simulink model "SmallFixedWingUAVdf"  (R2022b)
settings: Solver=ode4  StartTime=0  StopTime=stoptime  FixedStep=0.001  RelTol=1e-3  EnableMultiTasking=on
PreLoadFcn:
  | asbswarm_vehicledata; % load in workspace variables
PostLoadFcn:
  | open_system([gcs,'/MATLAB Animation Display/MATLAB',10,'Animation']);
InitFcn:
  | InitDatactrl
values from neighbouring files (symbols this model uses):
  env = struct    [InitDatactrl.m]
  F = Fattr + Frep    [APF.m]
  q = ix-1    [bspline_deboor.m]
  SenorSampleTime = 0.01    [InitDatactrl.m]
  sensors = struct    [InitDatactrl.m]
  uav = struct    [InitDatactrl.m]    (also in InitDatactrldf.m)
undefined symbols (not defined in the file or in its folder): Busy, Continuous, DiscIntNeverNeededParam, Dryden, Earth, Light, MIL, Newton, pa28, r, Raphson, sigbuilder_block, Wait, WGS84
libraries: simulink x37, aerolibactuator x10, sharedtransform x6, aerolibatmos2 x4, aerolibasang x4, aerolibwind2 x4, aerolibtransform2 x3, aerolibconvert2 x3, aerolibfltsims x2, shared6dof x2, aerolibnav x2, aerolibanimutils x1
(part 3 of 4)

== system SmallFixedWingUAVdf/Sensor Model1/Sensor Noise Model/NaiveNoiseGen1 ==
  Signal In : Inport
  Noise On : Inport  Port=2
  Add : Sum
  Band-Limited White Noise : simulink/Sources/Band-Limited White Noise  Cov=np  Ts=st  seed=ns
  Gain : Gain  Gain=ng
  Switch : Switch  Threshold=0.3
  Signal Out : Outport  VectorParamsAs1DForOutWhenUnconnected=off
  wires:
  Gain/1 -> Add/2
  Signal In/1 -> Add/1, Switch/3
  Switch/1 -> Signal Out/1
  Noise On/1 -> Switch/2
  Add/1 -> Switch/1
  Band-Limited White Noise/1 -> Gain/1

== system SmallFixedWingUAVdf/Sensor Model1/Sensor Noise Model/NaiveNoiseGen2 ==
  Signal In : Inport
  Noise On : Inport  Port=2
  Add : Sum
  Band-Limited White Noise : simulink/Sources/Band-Limited White Noise  Cov=np  Ts=st  seed=ns
  Gain : Gain  Gain=ng
  Switch : Switch  Threshold=0.3
  Signal Out : Outport  VectorParamsAs1DForOutWhenUnconnected=off
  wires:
  Gain/1 -> Add/2
  Signal In/1 -> Add/1, Switch/3
  Switch/1 -> Signal Out/1
  Noise On/1 -> Switch/2
  Add/1 -> Switch/1
  Band-Limited White Noise/1 -> Gain/1

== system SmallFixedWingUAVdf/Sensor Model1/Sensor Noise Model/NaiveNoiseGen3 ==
  Signal In : Inport
  Noise On : Inport  Port=2
  Add : Sum
  Band-Limited White Noise : simulink/Sources/Band-Limited White Noise  Cov=np  Ts=st  seed=ns
  Gain : Gain  Gain=ng
  Switch : Switch  Threshold=0.3
  Signal Out : Outport  VectorParamsAs1DForOutWhenUnconnected=off
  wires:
  Gain/1 -> Add/2
  Signal In/1 -> Add/1, Switch/3
  Switch/1 -> Signal Out/1
  Noise On/1 -> Switch/2
  Add/1 -> Switch/1
  Band-Limited White Noise/1 -> Gain/1

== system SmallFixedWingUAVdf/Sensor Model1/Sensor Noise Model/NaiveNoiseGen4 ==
  Signal In : Inport
  Noise On : Inport  Port=2
  Add : Sum
  Band-Limited White Noise : simulink/Sources/Band-Limited White Noise  Cov=np  Ts=st  seed=ns
  Gain : Gain  Gain=ng
  Switch : Switch  Threshold=0.3
  Signal Out : Outport  VectorParamsAs1DForOutWhenUnconnected=off
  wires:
  Gain/1 -> Add/2
  Signal In/1 -> Add/1, Switch/3
  Switch/1 -> Signal Out/1
  Noise On/1 -> Switch/2
  Add/1 -> Switch/1
  Band-Limited White Noise/1 -> Gain/1

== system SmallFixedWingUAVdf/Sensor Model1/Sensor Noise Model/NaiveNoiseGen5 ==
  Signal In : Inport
  Noise On : Inport  Port=2
  Add : Sum
  Band-Limited White Noise : simulink/Sources/Band-Limited White Noise  Cov=np  Ts=st  seed=ns
  Gain : Gain  Gain=ng
  Switch : Switch  Threshold=0.3
  Signal Out : Outport  VectorParamsAs1DForOutWhenUnconnected=off
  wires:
  Gain/1 -> Add/2
  Signal In/1 -> Add/1, Switch/3
  Switch/1 -> Signal Out/1
  Noise On/1 -> Switch/2
  Add/1 -> Switch/1
  Band-Limited White Noise/1 -> Gain/1

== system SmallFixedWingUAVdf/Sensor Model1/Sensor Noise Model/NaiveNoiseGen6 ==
  Signal In : Inport
  Noise On : Inport  Port=2
  Add : Sum
  Band-Limited White Noise : simulink/Sources/Band-Limited White Noise  Cov=np  Ts=st  seed=ns
  Gain : Gain  Gain=ng
  Switch : Switch  Threshold=0.3
  Signal Out : Outport  VectorParamsAs1DForOutWhenUnconnected=off
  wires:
  Gain/1 -> Add/2
  Signal In/1 -> Add/1, Switch/3
  Switch/1 -> Signal Out/1
  Noise On/1 -> Switch/2
  Add/1 -> Switch/1
  Band-Limited White Noise/1 -> Gain/1

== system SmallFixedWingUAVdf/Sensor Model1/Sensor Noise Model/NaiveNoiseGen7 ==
  Signal In : Inport
  Noise On : Inport  Port=2
  Add : Sum
  Band-Limited White Noise : simulink/Sources/Band-Limited White Noise  Cov=np  Ts=st  seed=ns
  Gain : Gain  Gain=ng
  Switch : Switch  Threshold=0.3
  Signal Out : Outport  VectorParamsAs1DForOutWhenUnconnected=off
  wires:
  Gain/1 -> Add/2
  Signal In/1 -> Add/1, Switch/3
  Switch/1 -> Signal Out/1
  Noise On/1 -> Switch/2
  Add/1 -> Switch/1
  Band-Limited White Noise/1 -> Gain/1

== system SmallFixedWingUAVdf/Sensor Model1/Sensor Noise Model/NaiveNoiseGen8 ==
  Signal In : Inport
  Noise On : Inport  Port=2
  Add : Sum
  Band-Limited White Noise : simulink/Sources/Band-Limited White Noise  Cov=np  Ts=st  seed=ns
  Gain : Gain  Gain=ng
  Switch : Switch  Threshold=0.3
  Signal Out : Outport  VectorParamsAs1DForOutWhenUnconnected=off
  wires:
  Gain/1 -> Add/2
  Signal In/1 -> Add/1, Switch/3
  Switch/1 -> Signal Out/1
  Noise On/1 -> Switch/2
  Add/1 -> Switch/1
  Band-Limited White Noise/1 -> Gain/1

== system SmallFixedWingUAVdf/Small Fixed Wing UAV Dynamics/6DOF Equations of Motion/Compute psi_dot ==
  Euler : Inport
  G : Inport  Port=2
  Mux1 : Mux  Inputs=2
  psidot : Fcn  Expr=(u[5]*sin(u[1])+u[6]*cos(u[1]))/cos(u[2])
  psi_dot : Outport  Unit=rad/S  VectorParamsAs1DForOutWhenUnconnected=off
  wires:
  G/1 -> Mux1/2
  psidot/1 -> psi_dot/1  "psi_dot"
  Mux1/1 -> psidot/1
  Euler/1 -> Mux1/1

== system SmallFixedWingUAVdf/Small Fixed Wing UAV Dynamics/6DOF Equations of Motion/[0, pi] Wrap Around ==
  Euler : Inport
  Compare To Zero : simulink/Logic and Bit Operations/Compare To Zero  relop=>=  OutDataTypeStr=uint8  ZeroCross=off
  Logical Operator : Logic  Operator=NOT  AllPortsSameDT=off  OutDataTypeStr=boolean
  Merge : Merge  InitialOutput=0
  Mux2 : Mux  Inputs=2
  Negative Yaw : Subsystem
  Positive Yaw : Subsystem
  Selector1 : Selector  InputPortWidth=3  IndexOptions=Index vector (dialog)  Indices=[1 2]  OutputSizes=1
  Selector2 : Selector  InputPortWidth=3  IndexOptions=Index vector (dialog)  Indices=[3]  OutputSizes=1
  Wrapped : Outport  VectorParamsAs1DForOutWhenUnconnected=off
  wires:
  Negative Yaw/1(yaw_wr) -> Merge/2
  Positive Yaw/1(yaw_wr) -> Merge/1
  Merge/1 -> Mux2/2
  Logical Operator/1 -> Negative Yaw/Enable
  Compare To Zero/1 -> Logical Operator/1, Positive Yaw/Enable
  Selector2/1 -> Negative Yaw/1(yaw), Positive Yaw/1(yaw), Compare To Zero/1
  Mux2/1 -> Wrapped/1
  Selector1/1 -> Mux2/1
  Euler/1 -> Selector1/1, Selector2/1

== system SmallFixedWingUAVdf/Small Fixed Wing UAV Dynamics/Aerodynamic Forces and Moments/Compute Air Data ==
  Vb : Inport  PortDimensions=3
  Rho : Inport  Port=2
  Bus Creator : BusCreator  Inputs=4
  Dynamic Pressure : aerolibasang/Dynamic Pressure
  "Incidence, Sideslip, & Airspeed" : aerolibasang/Incidence, Sideslip, & Airspeed
  AirData : Outport  VectorParamsAs1DForOutWhenUnconnected=off
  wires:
  Bus Creator/1 -> AirData/1
  "Incidence, Sideslip, & Airspeed"/1 -> Bus Creator/1  "alpha"
  Rho/1 -> Dynamic Pressure/2
  "Incidence, Sideslip, & Airspeed"/3 -> Bus Creator/3  "airpseed"
  Dynamic Pressure/1 -> Bus Creator/4  "q"
  Vb/1 -> "Incidence, Sideslip, & Airspeed"/1, Dynamic Pressure/1
  "Incidence, Sideslip, & Airspeed"/2 -> Bus Creator/2  "beta"

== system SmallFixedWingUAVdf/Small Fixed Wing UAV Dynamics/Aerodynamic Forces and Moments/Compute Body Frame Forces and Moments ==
  AirData : Inport
  CtrlSurfaces : Inport  Port=2
  p,q,r : Inport  Port=3
  Bus Selector : BusSelector  OutputSignals=alpha,beta
  Mux : Mux  Inputs=2
  Rotate FM to body frame : Subsystem
  Wind frame F& M : Subsystem
  F_b : Outport  Unit=kg*m/s^2  VectorParamsAs1DForOutWhenUnconnected=off
  M_b : Outport  Port=2  Unit=kg*m/s  VectorParamsAs1DForOutWhenUnconnected=off
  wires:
  Mux/1 -> Rotate FM to body frame/2(alpha_beta)
  Bus Selector/2 -> Mux/2  "<beta>"
  Bus Selector/1 -> Mux/1  "<alpha>"
  Wind frame F& M/1(FM_w) -> Rotate FM to body frame/1(FM_w)  "FM_W"
  p,q,r/1 -> Wind frame F& M/3(p,q,r)
  Rotate FM to body frame/2(M_b) -> M_b/1
  Rotate FM to body frame/1(F_b) -> F_b/1
  CtrlSurfaces/1 -> Wind frame F& M/2(CtrlSurfaces)
  AirData/1 -> Wind frame F& M/1(Airdata), Bus Selector/1

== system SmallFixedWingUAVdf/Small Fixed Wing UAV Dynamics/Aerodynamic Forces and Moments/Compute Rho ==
  Xe : Inport
  Gain : Gain  Gain=-1
  Get Z : Selector  InputPortWidth=3  IndexOptions=Index vector (dialog)  Indices=[3]  OutputSizes=[(-2)]
  ISA Atmosphere Model1 : aerolibatmos2/ISA Atmosphere Model  custom=on  g=env.ISA_g  gamma=1.4  R=env.ISA_R  L=env.ISA_lapse  h_trop=11000  h_strat=20000  rho0=env.ISA_rho0  P0=env.ISA_P0  T0=env.ISA_T0  h0=0
  Terminator : Terminator
  Terminator1 : Terminator
  Terminator2 : Terminator
  Transfer Fcn : TransferFcn  Denominator=[.01 1]
  Rho : Outport  VectorParamsAs1DForOutWhenUnconnected=off
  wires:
  ISA Atmosphere Model1/2 -> Terminator1/1
  ISA Atmosphere Model1/1 -> Terminator/1  "OAT"
  Gain/1 -> ISA Atmosphere Model1/1
  Get Z/1 -> Transfer Fcn/1
  Transfer Fcn/1 -> Gain/1
  ISA Atmosphere Model1/3 -> Terminator2/1  "static"
  Xe/1 -> Get Z/1
  ISA Atmosphere Model1/4 -> Rho/1

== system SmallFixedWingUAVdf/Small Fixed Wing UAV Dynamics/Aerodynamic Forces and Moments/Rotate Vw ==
  Vw : Inport
  Euler : Inport  Port=2
  RL2B : Subsystem
  RL2B * Vw : Product  Multiplication=Matrix(*)  InputSameDT=on  SaturateOnIntegerOverflow=on
  Vb : Outport  Unit=m/s  VectorParamsAs1DForOutWhenUnconnected=off
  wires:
  RL2B * Vw/1 -> Vb/1
  Vw/1 -> RL2B * Vw/2
  RL2B/1(RL2B) -> RL2B * Vw/1
  Euler/1 -> RL2B/1(Euler)

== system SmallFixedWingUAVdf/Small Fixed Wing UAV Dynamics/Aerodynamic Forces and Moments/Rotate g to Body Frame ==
  Euler : Inport
  Gravity Force : Inport  Port=2  PortDimensions=3
  Product1 : Product  Multiplication=Matrix(*)  InputSameDT=on  SaturateOnIntegerOverflow=on
  RL2B : Subsystem
  g_b : Outport  Unit=kg*m/s^2  VectorParamsAs1DForOutWhenUnconnected=off
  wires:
  Gravity Force/1 -> Product1/2
  Euler/1 -> RL2B/1(Euler)
  Product1/1 -> g_b/1
  RL2B/1(RL2B) -> Product1/1

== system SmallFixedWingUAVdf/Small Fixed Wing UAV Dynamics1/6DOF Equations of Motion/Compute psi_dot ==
  Euler : Inport
  G : Inport  Port=2
  Mux1 : Mux  Inputs=2
  psidot : Fcn  Expr=(u[5]*sin(u[1])+u[6]*cos(u[1]))/cos(u[2])
  psi_dot : Outport  Unit=rad/S  VectorParamsAs1DForOutWhenUnconnected=off
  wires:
  G/1 -> Mux1/2
  psidot/1 -> psi_dot/1  "psi_dot"
  Mux1/1 -> psidot/1
  Euler/1 -> Mux1/1

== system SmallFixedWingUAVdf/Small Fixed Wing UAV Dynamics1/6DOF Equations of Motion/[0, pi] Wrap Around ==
  Euler : Inport
  Compare To Zero : simulink/Logic and Bit Operations/Compare To Zero  relop=>=  OutDataTypeStr=uint8  ZeroCross=off
  Logical Operator : Logic  Operator=NOT  AllPortsSameDT=off  OutDataTypeStr=boolean
  Merge : Merge  InitialOutput=0
  Mux2 : Mux  Inputs=2
  Negative Yaw : Subsystem
  Positive Yaw : Subsystem
  Selector1 : Selector  InputPortWidth=3  IndexOptions=Index vector (dialog)  Indices=[1 2]  OutputSizes=1
  Selector2 : Selector  InputPortWidth=3  IndexOptions=Index vector (dialog)  Indices=[3]  OutputSizes=1
  Wrapped : Outport  VectorParamsAs1DForOutWhenUnconnected=off
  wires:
  Negative Yaw/1(yaw_wr) -> Merge/2
  Positive Yaw/1(yaw_wr) -> Merge/1
  Merge/1 -> Mux2/2
  Logical Operator/1 -> Negative Yaw/Enable
  Compare To Zero/1 -> Logical Operator/1, Positive Yaw/Enable
  Selector2/1 -> Negative Yaw/1(yaw), Positive Yaw/1(yaw), Compare To Zero/1
  Mux2/1 -> Wrapped/1
  Selector1/1 -> Mux2/1
  Euler/1 -> Selector1/1, Selector2/1

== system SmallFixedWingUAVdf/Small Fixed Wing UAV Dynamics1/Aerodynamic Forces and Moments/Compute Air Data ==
  Vb : Inport  PortDimensions=3
  Rho : Inport  Port=2
  Bus Creator : BusCreator  Inputs=4
  Dynamic Pressure : aerolibasang/Dynamic Pressure
  "Incidence, Sideslip, & Airspeed" : aerolibasang/Incidence, Sideslip, & Airspeed
  AirData : Outport  VectorParamsAs1DForOutWhenUnconnected=off
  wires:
  Bus Creator/1 -> AirData/1  "AirData"
  "Incidence, Sideslip, & Airspeed"/1 -> Bus Creator/1  "alpha"
  Rho/1 -> Dynamic Pressure/2
  "Incidence, Sideslip, & Airspeed"/3 -> Bus Creator/3  "airpseed"
  Dynamic Pressure/1 -> Bus Creator/4  "q"
  Vb/1 -> "Incidence, Sideslip, & Airspeed"/1, Dynamic Pressure/1
  "Incidence, Sideslip, & Airspeed"/2 -> Bus Creator/2  "beta"

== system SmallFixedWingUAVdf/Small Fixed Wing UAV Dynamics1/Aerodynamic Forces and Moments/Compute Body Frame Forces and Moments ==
  AirData : Inport
  CtrlSurfaces : Inport  Port=2
  p,q,r : Inport  Port=3
  Bus Selector : BusSelector  OutputSignals=alpha,beta
  Mux : Mux  Inputs=2
  Rotate FM to body frame : Subsystem
  Wind frame F& M : Subsystem
  F_b : Outport  Unit=kg*m/s^2  VectorParamsAs1DForOutWhenUnconnected=off
  M_b : Outport  Port=2  Unit=kg*m/s  VectorParamsAs1DForOutWhenUnconnected=off
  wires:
  Mux/1 -> Rotate FM to body frame/2(alpha_beta)
  Bus Selector/2 -> Mux/2  "<beta>"
  Bus Selector/1 -> Mux/1  "<alpha>"
  Wind frame F& M/1(FM_w) -> Rotate FM to body frame/1(FM_w)  "FM_W"
  p,q,r/1 -> Wind frame F& M/3(p,q,r)
  Rotate FM to body frame/2(M_b) -> M_b/1
  Rotate FM to body frame/1(F_b) -> F_b/1
  CtrlSurfaces/1 -> Wind frame F& M/2(CtrlSurfaces)
  AirData/1 -> Wind frame F& M/1(Airdata), Bus Selector/1

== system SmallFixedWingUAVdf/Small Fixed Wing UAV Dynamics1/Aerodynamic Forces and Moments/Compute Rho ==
  Xe : Inport
  Gain : Gain  Gain=-1
  Get Z : Selector  InputPortWidth=3  IndexOptions=Index vector (dialog)  Indices=[3]  OutputSizes=[(-2)]
  ISA Atmosphere Model1 : aerolibatmos2/ISA Atmosphere Model  custom=on  g=env.ISA_g  gamma=1.4  R=env.ISA_R  L=env.ISA_lapse  h_trop=11000  h_strat=20000  rho0=env.ISA_rho0  P0=env.ISA_P0  T0=env.ISA_T0  h0=0
  Terminator : Terminator
  Terminator1 : Terminator
  Terminator2 : Terminator
  Transfer Fcn : TransferFcn  Denominator=[.01 1]
  Rho : Outport  VectorParamsAs1DForOutWhenUnconnected=off
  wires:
  ISA Atmosphere Model1/2 -> Terminator1/1
  ISA Atmosphere Model1/1 -> Terminator/1  "OAT"
  Gain/1 -> ISA Atmosphere Model1/1
  Get Z/1 -> Transfer Fcn/1
  Transfer Fcn/1 -> Gain/1
  ISA Atmosphere Model1/3 -> Terminator2/1  "static"
  Xe/1 -> Get Z/1
  ISA Atmosphere Model1/4 -> Rho/1

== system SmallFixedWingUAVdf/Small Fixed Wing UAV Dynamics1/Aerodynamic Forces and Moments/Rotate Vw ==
  Vw : Inport
  Euler : Inport  Port=2
  RL2B : Subsystem
  RL2B * Vw : Product  Multiplication=Matrix(*)  InputSameDT=on  SaturateOnIntegerOverflow=on
  Vb : Outport  Unit=m/s  VectorParamsAs1DForOutWhenUnconnected=off
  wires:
  RL2B * Vw/1 -> Vb/1
  Vw/1 -> RL2B * Vw/2
  RL2B/1(RL2B) -> RL2B * Vw/1
  Euler/1 -> RL2B/1(Euler)

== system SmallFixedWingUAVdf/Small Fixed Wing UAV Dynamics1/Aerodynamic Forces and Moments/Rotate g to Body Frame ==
  Euler : Inport
  Gravity Force : Inport  Port=2  PortDimensions=3
  Product1 : Product  Multiplication=Matrix(*)  InputSameDT=on  SaturateOnIntegerOverflow=on
  RL2B : Subsystem
  g_b : Outport  Unit=kg*m/s^2  VectorParamsAs1DForOutWhenUnconnected=off
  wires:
  Gravity Force/1 -> Product1/2
  Euler/1 -> RL2B/1(Euler)
  Product1/1 -> g_b/1
  RL2B/1(RL2B) -> Product1/1

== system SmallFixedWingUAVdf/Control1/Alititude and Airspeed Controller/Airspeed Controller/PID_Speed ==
  x : Inport
  reset_i : Inport  Port=2
  Derivative Gain : Gain  DisableCoverage=on  Gain=0  ParamMin=-100  ParamMax=100  OutMin=-100  OutMax=100
  Discrete Derivative : simulink/Discrete/Discrete Derivative  gainval=1.0  ICPrevScaledInput=0.0  OutMin=[]  OutMax=[]  OutDataType=fixdt(1, 16)  OutScaling=2^-10  DoSatur=off
  Discrete-Time Integrator : DiscreteIntegrator  ExternalReset=either  SampleTime=-1  UpperSaturationLimit=0.3  LowerSaturationLimit=-0.3  ICPrevOutput=DiscIntNeverNeededParam  ICPrevScaledInput=DiscIntNeverNeededParam
  Gain : Gain  Gain=0.5
  Integral Gain : Gain  DisableCoverage=on  Gain=0.13
  Sum : Sum  Inputs=+++
  y : Outport  InitialOutput=0  VectorParamsAs1DForOutWhenUnconnected=off
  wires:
  reset_i/1 -> Discrete-Time Integrator/2
  Discrete-Time Integrator/1 -> Sum/2
  Discrete Derivative/1 -> Sum/3
  Sum/1 -> y/1
  Gain/1 -> Sum/1
  Derivative Gain/1 -> Discrete Derivative/1
  Integral Gain/1 -> Discrete-Time Integrator/1
  x/1 -> Derivative Gain/1, Integral Gain/1, Gain/1

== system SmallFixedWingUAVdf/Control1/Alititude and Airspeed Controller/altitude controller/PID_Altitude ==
  x : Inport
  reset_i : Inport  Port=2
  Derivative Gain : Gain  DisableCoverage=on  Gain=0  ParamMin=-100  ParamMax=100  OutMin=-100  OutMax=100
  Discrete Derivative : simulink/Discrete/Discrete Derivative  gainval=1.0  ICPrevScaledInput=0.0  OutMin=[]  OutMax=[]  OutDataType=fixdt(1, 16)  OutScaling=2^-10  DoSatur=off
  Discrete-Time Integrator : DiscreteIntegrator  ExternalReset=either  SampleTime=-1  ICPrevOutput=DiscIntNeverNeededParam  ICPrevScaledInput=DiscIntNeverNeededParam
  Gain : Gain  Gain=0.055
  Integral Gain : Gain  DisableCoverage=on  Gain=0
  Sum : Sum  Inputs=+++
  y : Outport  InitialOutput=0  VectorParamsAs1DForOutWhenUnconnected=off
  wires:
  x/1 -> Gain/1, Integral Gain/1, Derivative Gain/1
  Integral Gain/1 -> Discrete-Time Integrator/1
  Derivative Gain/1 -> Discrete Derivative/1
  Gain/1 -> Sum/1
  Sum/1 -> y/1
  Discrete Derivative/1 -> Sum/3
  Discrete-Time Integrator/1 -> Sum/2
  reset_i/1 -> Discrete-Time Integrator/2

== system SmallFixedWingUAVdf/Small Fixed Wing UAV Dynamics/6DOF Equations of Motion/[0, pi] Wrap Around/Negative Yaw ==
  yaw : Inport
  Enable : EnablePort
  Abs : Abs
  Constant1 : Constant  Value=2*pi
  Constant2 : Constant  Value=2*pi
  Math Function : Math  Operator=mod  SignedPower=on
  Sum : Sum  Inputs=|-+
  yaw_wr : Outport  VectorParamsAs1DForOutWhenUnconnected=off
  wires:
  Sum/1 -> yaw_wr/1
  Constant2/1 -> Sum/2
  Abs/1 -> Math Function/1
  Math Function/1 -> Sum/1
  Constant1/1 -> Math Function/2
  yaw/1 -> Abs/1

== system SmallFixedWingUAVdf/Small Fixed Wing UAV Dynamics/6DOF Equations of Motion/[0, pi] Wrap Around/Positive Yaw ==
  yaw : Inport
  Enable : EnablePort
  Constant1 : Constant  Value=2*pi
  Math Function : Math  Operator=mod  SignedPower=on
  yaw_wr : Outport  VectorParamsAs1DForOutWhenUnconnected=off
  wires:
  Math Function/1 -> yaw_wr/1
  Constant1/1 -> Math Function/2
  yaw/1 -> Math Function/1

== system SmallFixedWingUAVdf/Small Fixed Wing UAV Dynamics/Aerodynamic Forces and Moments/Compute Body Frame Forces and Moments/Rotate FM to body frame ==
  FM_w : Inport
  alpha_beta : Inport  Port=2
  Forces : Selector  InputPortWidth=6  IndexOptions=Index vector (dialog)  Indices=[1 2 3]  OutputSizes=[(-2)]
  Moments : Selector  InputPortWidth=6  IndexOptions=Index vector (dialog)  Indices=[4 5 6]  OutputSizes=[(-2)]
  Rotate Forces : Subsystem
  Rotate Moments : Subsystem
  F_b : Outport  VectorParamsAs1DForOutWhenUnconnected=off
  M_b : Outport  Port=2  VectorParamsAs1DForOutWhenUnconnected=off
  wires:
  alpha_beta/1 -> Rotate Forces/2(alpha_beta), Rotate Moments/1(alpha_beta)
  Moments/1 -> Rotate Moments/2(M_w)
  FM_w/1 -> Moments/1, Forces/1
  Forces/1 -> Rotate Forces/1(F_w)
  Rotate Moments/1(M_b) -> M_b/1
  Rotate Forces/1(F_b) -> F_b/1

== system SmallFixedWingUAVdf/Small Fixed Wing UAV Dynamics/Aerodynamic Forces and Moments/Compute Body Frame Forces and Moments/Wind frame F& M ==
  Airdata : Inport
  CtrlSurfaces : Inport  Port=2
  p,q,r : Inport  Port=3
  Bus Creator1 : BusCreator  Inputs=2
  Bus Selector1 : BusSelector  OutputSignals=dA,dR
  Bus Selector2 : BusSelector  OutputSignals=dE,dF
  Bus Selector6 : BusSelector  OutputSignals=beta,airpseed
  Bus Selector7 : BusSelector  OutputSignals=alpha,airpseed
  Get Forces and Moments : Subsystem
  Lateral Channel : Subsystem
  Longitudinal Channel : Subsystem
  FM_w : Outport  PortDimensions=6  VectorParamsAs1DForOutWhenUnconnected=off
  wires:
  Get Forces and Moments/1(FM_w) -> FM_w/1
  Bus Creator1/1 -> Get Forces and Moments/2(AeroCoeffs)
  Bus Selector7/2 -> Longitudinal Channel/2(Airpseed)  "<airpseed>"
  Bus Selector7/1 -> Longitudinal Channel/1(alpha)  "<alpha>"
  Bus Selector6/2 -> Lateral Channel/2(Airspeed)  "<airpseed>"
  Bus Selector6/1 -> Lateral Channel/1(beta)  "<beta>"
  Airdata/1 -> Bus Selector6/1, Bus Selector7/1, Get Forces and Moments/1(Airdata)
  Bus Selector2/2 -> Longitudinal Channel/4(dF)  "<dF>"
  Bus Selector2/1 -> Longitudinal Channel/3(dE)  "<dE>"
  Bus Selector1/2 -> Lateral Channel/4(dR)  "<dR>"
  Bus Selector1/1 -> Lateral Channel/3(dA)  "<dA>"
  CtrlSurfaces/1 -> Bus Selector1/1, Bus Selector2/1
  p,q,r/1 -> Lateral Channel/5(p,q,r), Longitudinal Channel/5(p,q,r)
  Lateral Channel/1(Lateral) -> Bus Creator1/1
  Longitudinal Channel/1(Longitudinal) -> Bus Creator1/2

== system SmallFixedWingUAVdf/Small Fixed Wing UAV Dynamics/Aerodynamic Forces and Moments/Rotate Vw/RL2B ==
  Euler : Inport
  Rotation Angles to Direction Cosine Matrix : sharedtransform/Rotation Angles to Direction Cosine Matrix  rotationOrder=ZYX  aMode=aMode
  Selector : Selector  InputPortWidth=3  IndexOptions=Index vector (dialog)  Indices=[3 2 1]  OutputSizes=1
  RL2B : Outport  VectorParamsAs1DForOutWhenUnconnected=off
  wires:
  Rotation Angles to Direction Cosine Matrix/1 -> RL2B/1
  Euler/1 -> Selector/1
  Selector/1 -> Rotation Angles to Direction Cosine Matrix/1

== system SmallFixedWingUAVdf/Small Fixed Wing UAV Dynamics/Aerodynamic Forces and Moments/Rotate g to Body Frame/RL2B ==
  Euler : Inport
  Rotation Angles to Direction Cosine Matrix : sharedtransform/Rotation Angles to Direction Cosine Matrix  rotationOrder=ZYX  aMode=aMode
  Selector : Selector  InputPortWidth=3  IndexOptions=Index vector (dialog)  Indices=[3 2 1]  OutputSizes=1
  RL2B : Outport  VectorParamsAs1DForOutWhenUnconnected=off
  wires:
  Rotation Angles to Direction Cosine Matrix/1 -> RL2B/1
  Euler/1 -> Selector/1
  Selector/1 -> Rotation Angles to Direction Cosine Matrix/1

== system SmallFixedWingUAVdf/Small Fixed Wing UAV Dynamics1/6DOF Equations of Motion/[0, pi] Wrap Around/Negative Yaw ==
  yaw : Inport
  Enable : EnablePort
  Abs : Abs
  Constant1 : Constant  Value=2*pi
  Constant2 : Constant  Value=2*pi
  Math Function : Math  Operator=mod  SignedPower=on
  Sum : Sum  Inputs=|-+
  yaw_wr : Outport  VectorParamsAs1DForOutWhenUnconnected=off
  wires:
  Sum/1 -> yaw_wr/1
  Constant2/1 -> Sum/2
  Abs/1 -> Math Function/1
  Math Function/1 -> Sum/1
  Constant1/1 -> Math Function/2
  yaw/1 -> Abs/1

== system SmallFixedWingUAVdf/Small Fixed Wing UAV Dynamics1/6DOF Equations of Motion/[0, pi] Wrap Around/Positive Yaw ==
  yaw : Inport
  Enable : EnablePort
  Constant1 : Constant  Value=2*pi
  Math Function : Math  Operator=mod  SignedPower=on
  yaw_wr : Outport  VectorParamsAs1DForOutWhenUnconnected=off
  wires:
  Math Function/1 -> yaw_wr/1
  Constant1/1 -> Math Function/2
  yaw/1 -> Math Function/1

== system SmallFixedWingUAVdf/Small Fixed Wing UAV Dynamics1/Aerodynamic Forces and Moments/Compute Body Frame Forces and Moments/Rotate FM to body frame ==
  FM_w : Inport
  alpha_beta : Inport  Port=2
  Forces : Selector  InputPortWidth=6  IndexOptions=Index vector (dialog)  Indices=[1 2 3]  OutputSizes=[(-2)]
  Moments : Selector  InputPortWidth=6  IndexOptions=Index vector (dialog)  Indices=[4 5 6]  OutputSizes=[(-2)]
  Rotate Forces : Subsystem
  Rotate Moments : Subsystem
  F_b : Outport  VectorParamsAs1DForOutWhenUnconnected=off
  M_b : Outport  Port=2  VectorParamsAs1DForOutWhenUnconnected=off
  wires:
  alpha_beta/1 -> Rotate Forces/2(alpha_beta), Rotate Moments/1(alpha_beta)
  Moments/1 -> Rotate Moments/2(M_w)
  FM_w/1 -> Moments/1, Forces/1
  Forces/1 -> Rotate Forces/1(F_w)
  Rotate Moments/1(M_b) -> M_b/1
  Rotate Forces/1(F_b) -> F_b/1

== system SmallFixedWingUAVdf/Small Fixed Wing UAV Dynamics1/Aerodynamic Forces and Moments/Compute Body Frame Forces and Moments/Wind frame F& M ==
  Airdata : Inport
  CtrlSurfaces : Inport  Port=2
  p,q,r : Inport  Port=3
  Bus Creator1 : BusCreator  Inputs=2
  Bus Selector1 : BusSelector  OutputSignals=dA,dR
  Bus Selector2 : BusSelector  OutputSignals=dE,dF
  Bus Selector6 : BusSelector  OutputSignals=beta,airpseed
  Bus Selector7 : BusSelector  OutputSignals=alpha,airpseed
  Get Forces and Moments : Subsystem
  Lateral Channel : Subsystem
  Longitudinal Channel : Subsystem
  FM_w : Outport  PortDimensions=6  VectorParamsAs1DForOutWhenUnconnected=off
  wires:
  Get Forces and Moments/1(FM_w) -> FM_w/1
  Bus Creator1/1 -> Get Forces and Moments/2(AeroCoeffs)
  Bus Selector7/2 -> Longitudinal Channel/2(Airpseed)  "<airpseed>"
  Bus Selector7/1 -> Longitudinal Channel/1(alpha)  "<alpha>"
  Bus Selector6/2 -> Lateral Channel/2(Airspeed)  "<airpseed>"
  Bus Selector6/1 -> Lateral Channel/1(beta)  "<beta>"
  Airdata/1 -> Get Forces and Moments/1(Airdata), Bus Selector7/1, Bus Selector6/1
  Bus Selector2/2 -> Longitudinal Channel/4(dF)  "<dF>"
  Bus Selector2/1 -> Longitudinal Channel/3(dE)  "<dE>"
  Bus Selector1/2 -> Longitudinal Channel/6(dR), Lateral Channel/4(dR)  "<dR>"
  Bus Selector1/1 -> Lateral Channel/3(dA)  "<dA>"
  CtrlSurfaces/1 -> Bus Selector2/1, Bus Selector1/1
  p,q,r/1 -> Lateral Channel/5(p,q,r), Longitudinal Channel/5(p,q,r)
  Lateral Channel/1(Lateral) -> Bus Creator1/1
  Longitudinal Channel/1(Longitudinal) -> Bus Creator1/2

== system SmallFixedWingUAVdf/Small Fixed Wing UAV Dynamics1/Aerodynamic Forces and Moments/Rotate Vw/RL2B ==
  Euler : Inport
  Rotation Angles to Direction Cosine Matrix : sharedtransform/Rotation Angles to Direction Cosine Matrix  rotationOrder=ZYX  aMode=aMode
  Selector : Selector  InputPortWidth=3  IndexOptions=Index vector (dialog)  Indices=[3 2 1]  OutputSizes=1
  RL2B : Outport  VectorParamsAs1DForOutWhenUnconnected=off
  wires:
  Rotation Angles to Direction Cosine Matrix/1 -> RL2B/1
  Euler/1 -> Selector/1
  Selector/1 -> Rotation Angles to Direction Cosine Matrix/1

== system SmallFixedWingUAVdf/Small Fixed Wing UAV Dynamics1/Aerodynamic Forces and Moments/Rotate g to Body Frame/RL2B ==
  Euler : Inport
  Rotation Angles to Direction Cosine Matrix : sharedtransform/Rotation Angles to Direction Cosine Matrix  rotationOrder=ZYX  aMode=aMode
  Selector : Selector  InputPortWidth=3  IndexOptions=Index vector (dialog)  Indices=[3 2 1]  OutputSizes=1
  RL2B : Outport  VectorParamsAs1DForOutWhenUnconnected=off
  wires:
  Rotation Angles to Direction Cosine Matrix/1 -> RL2B/1
  Euler/1 -> Selector/1
  Selector/1 -> Rotation Angles to Direction Cosine Matrix/1

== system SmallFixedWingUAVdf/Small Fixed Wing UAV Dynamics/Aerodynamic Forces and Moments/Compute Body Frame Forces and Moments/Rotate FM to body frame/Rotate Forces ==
  F_w : Inport
  alpha_beta : Inport  Port=2
  Product2 : Product  Multiplication=Matrix(*)  SaturateOnIntegerOverflow=on
  RB2W : Subsystem
  RW2B : Math  Operator=transpose  SignedPower=on
  F_b : Outport  PortDimensions=3  VectorParamsAs1DForOutWhenUnconnected=off
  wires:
  RW2B/1 -> Product2/1
  F_w/1 -> Product2/2
  Product2/1 -> F_b/1
  alpha_beta/1 -> RB2W/1(aoa beta)
  RB2W/1(Rw2b) -> RW2B/1

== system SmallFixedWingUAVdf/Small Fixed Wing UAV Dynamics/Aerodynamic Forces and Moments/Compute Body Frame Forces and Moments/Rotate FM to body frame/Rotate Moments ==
  alpha_beta : Inport
  M_w : Inport  Port=2
  Product2 : Product  Multiplication=Matrix(*)  SaturateOnIntegerOverflow=on
  RB2W : Subsystem
  RW2B : Math  Operator=transpose  SignedPower=on
  M_b : Outport  PortDimensions=3  VectorParamsAs1DForOutWhenUnconnected=off
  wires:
  RW2B/1 -> Product2/1
  RB2W/1(Rw2b) -> RW2B/1
  alpha_beta/1 -> RB2W/1(aoa beta)
  Product2/1 -> M_b/1
  M_w/1 -> Product2/2

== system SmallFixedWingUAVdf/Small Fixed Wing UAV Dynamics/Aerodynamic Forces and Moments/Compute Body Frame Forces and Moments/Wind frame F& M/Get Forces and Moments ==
  Airdata : Inport
  AeroCoeffs : Inport  Port=2
  Bus Selector : BusSelector  OutputSignals=signal2.CD,signal1.CY,signal2.CL
  Bus Selector3 : BusSelector  OutputSignals=signal1.Cl,signal1.Cn
  Bus Selector4 : BusSelector  OutputSignals=signal2.Cm
  Bus Selector5 : BusSelector  OutputSignals=q
  Fx_a(Drag) : Product  Inputs=**  SaturateOnIntegerOverflow=on
  Fy_a(Side) : Product  SaturateOnIntegerOverflow=on
  Fz_a(Lift) : Product  SaturateOnIntegerOverflow=on
  Mux : Mux  Inputs=6
  Mx_a : Product  Inputs=3  SaturateOnIntegerOverflow=on
  My_a : Product  Inputs=3  SaturateOnIntegerOverflow=on
  Mz_a : Product  Inputs=3  SaturateOnIntegerOverflow=on
  Product1 : Product  Inputs=3  SaturateOnIntegerOverflow=on
  chord : Constant  Value=uav.geometry.chord  VectorParams1D=off
  span : Constant  Value=uav.geometry.span  VectorParams1D=off
  span1 : Constant  Value=uav.geometry.span  VectorParams1D=off
  span2 : Constant  Value=uav.geometry.chord  VectorParams1D=off
  FM_w : Outport  VectorParamsAs1DForOutWhenUnconnected=off
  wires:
  Mx_a/1 -> Mux/4  "Mx_a"
  Bus Selector/2 -> Fy_a(Side)/1  "<CY>"
  Bus Selector4/1 -> My_a/1  "<Cm>"
  span2/1 -> Product1/3
  Fx_a(Drag)/1 -> Mux/1  "Fx_a"
  Bus Selector/1 -> Fx_a(Drag)/1  "<CD>"
  AeroCoeffs/1 -> Bus Selector/1, Bus Selector4/1, Bus Selector3/1
  My_a/1 -> Mux/5  "My_a"
  Fz_a(Lift)/1 -> Mux/3  "Fz_a"
  Mz_a/1 -> Mux/6  "Mz_a"
  Airdata/1 -> Bus Selector5/1
  chord/1 -> My_a/3
  span/1 -> Mz_a/3, Mx_a/3
  Fy_a(Side)/1 -> Mux/2  "Fy_a"
  Mux/1 -> FM_w/1
  Bus Selector3/2 -> Mz_a/1  "<Cn>"
  Bus Selector/3 -> Fz_a(Lift)/1  "<CL>"
  Product1/1 -> Fx_a(Drag)/2, Fy_a(Side)/2, Fz_a(Lift)/2, Mx_a/2, My_a/2, Mz_a/2  "qS"
  span1/1 -> Product1/2
  Bus Selector3/1 -> Mx_a/1  "<Cl>"
  Bus Selector5/1 -> Product1/1  "<q>"

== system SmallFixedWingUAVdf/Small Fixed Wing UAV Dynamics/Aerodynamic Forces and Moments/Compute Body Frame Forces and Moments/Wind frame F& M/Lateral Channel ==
  beta : Inport
  Airspeed : Inport  Port=2
  dA : Inport  Port=3
  dR : Inport  Port=4
  p,q,r : Inport  Port=5
  Bus Creator : BusCreator  Inputs=3
  CY : Subsystem
  Cl : Subsystem
  Cn : Subsystem
  Lateral : Outport  VectorParamsAs1DForOutWhenUnconnected=off
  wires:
  Cl/1(Cl) -> Bus Creator/2  "Cl"
  p,q,r/1 -> Cn/4(p,q,r), Cl/4(p,q,r)
  Airspeed/1 -> Cn/5(Airspeed), Cl/5(Airspeed)
  dR/1 -> CY/2(dR), Cl/3(dR), Cn/3(dR)
  dA/1 -> Cl/2(dA), Cn/2(dA)
  beta/1 -> CY/1(beta), Cl/1(beta), Cn/1(beta)
  Cn/1(Cn) -> Bus Creator/3  "Cn"
  CY/1(CY) -> Bus Creator/1  "CY"
  Bus Creator/1 -> Lateral/1

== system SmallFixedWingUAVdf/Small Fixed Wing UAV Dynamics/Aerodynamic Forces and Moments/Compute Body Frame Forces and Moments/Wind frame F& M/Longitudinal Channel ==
  alpha : Inport
  Airpseed : Inport  Port=2
  dE : Inport  Port=3
  dF : Inport  Port=4
  p,q,r : Inport  Port=5
  Bus Creator : BusCreator  Inputs=3
  CD : Subsystem
  CL : Subsystem
  Cm : Subsystem
  Transfer Fcn : TransferFcn  Numerator=[1 0]  Denominator=[0.1 1]
  Y-down : Gain  Gain=-1  SaturateOnIntegerOverflow=on
  Longitudinal : Outport  VectorParamsAs1DForOutWhenUnconnected=off
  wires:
  Transfer Fcn/1 -> CL/2(alpha_dot)
  Airpseed/1 -> CL/6(Airspeed)
  p,q,r/1 -> Cm/4(p,q,r), CL/5(p,q,r)
  dF/1 -> Cm/3(dF), CL/4(dF)
  Bus Creator/1 -> Longitudinal/1
  Cm/1(Cm) -> Bus Creator/3  "Cm"
  CL/1(CL) -> CD/1(CL), Y-down/1
  dE/1 -> Cm/2(dE), CL/3(dE)
  Y-down/1 -> Bus Creator/2  "CL"
  CD/1(CD) -> Bus Creator/1  "CD"
  alpha/1 -> Transfer Fcn/1, Cm/1(alpha), CL/1(alpha)

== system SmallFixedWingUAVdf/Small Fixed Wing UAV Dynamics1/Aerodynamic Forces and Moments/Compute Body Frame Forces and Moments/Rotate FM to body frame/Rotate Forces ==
  F_w : Inport
  alpha_beta : Inport  Port=2
  Product2 : Product  Multiplication=Matrix(*)  SaturateOnIntegerOverflow=on
  RB2W : Subsystem
  RW2B : Math  Operator=transpose  SignedPower=on
  F_b : Outport  PortDimensions=3  VectorParamsAs1DForOutWhenUnconnected=off
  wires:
  RW2B/1 -> Product2/1
  F_w/1 -> Product2/2
  Product2/1 -> F_b/1
  alpha_beta/1 -> RB2W/1(aoa beta)
  RB2W/1(Rw2b) -> RW2B/1

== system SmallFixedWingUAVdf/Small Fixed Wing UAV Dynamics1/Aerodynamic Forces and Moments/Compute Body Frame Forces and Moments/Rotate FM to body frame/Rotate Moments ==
  alpha_beta : Inport
  M_w : Inport  Port=2
  Product2 : Product  Multiplication=Matrix(*)  SaturateOnIntegerOverflow=on
  RB2W : Subsystem
  RW2B : Math  Operator=transpose  SignedPower=on
  M_b : Outport  PortDimensions=3  VectorParamsAs1DForOutWhenUnconnected=off
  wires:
  RW2B/1 -> Product2/1
  RB2W/1(Rw2b) -> RW2B/1
  alpha_beta/1 -> RB2W/1(aoa beta)
  Product2/1 -> M_b/1
  M_w/1 -> Product2/2

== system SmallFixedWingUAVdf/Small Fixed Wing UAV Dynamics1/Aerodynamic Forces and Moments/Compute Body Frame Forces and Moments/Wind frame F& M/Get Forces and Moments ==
  Airdata : Inport
  AeroCoeffs : Inport  Port=2
  Bus Selector : BusSelector  OutputSignals=signal2.CD,signal1.CY,signal2.CL
  Bus Selector3 : BusSelector  OutputSignals=signal1.Cl,signal1.Cn
  Bus Selector4 : BusSelector  OutputSignals=signal2.Cm
  Bus Selector5 : BusSelector  OutputSignals=q
  Fx_a(Drag) : Product  Inputs=**  SaturateOnIntegerOverflow=on
  Fy_a(Side) : Product  SaturateOnIntegerOverflow=on
  Fz_a(Lift) : Product  SaturateOnIntegerOverflow=on
  Mux : Mux  Inputs=6
  Mx_a : Product  Inputs=3  SaturateOnIntegerOverflow=on
  My_a : Product  Inputs=3  SaturateOnIntegerOverflow=on
  Mz_a : Product  Inputs=3  SaturateOnIntegerOverflow=on
  Product1 : Product  SaturateOnIntegerOverflow=on
  chord : Constant  Value=uav.geometry.chord  VectorParams1D=off
  span : Constant  Value=uav.geometry.span  VectorParams1D=off
  span1 : Constant  Value=uav.geometry.S  VectorParams1D=off
  FM_w : Outport  VectorParamsAs1DForOutWhenUnconnected=off
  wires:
  Mx_a/1 -> Mux/4  "Mx_a"
  Bus Selector/2 -> Fy_a(Side)/1  "<CY>"
  Bus Selector4/1 -> My_a/1  "<Cm>"
  Fx_a(Drag)/1 -> Mux/1  "Fx_a"
  Bus Selector/1 -> Fx_a(Drag)/1  "<CD>"
  AeroCoeffs/1 -> Bus Selector/1, Bus Selector4/1, Bus Selector3/1
  My_a/1 -> Mux/5  "My_a"
  Fz_a(Lift)/1 -> Mux/3  "Fz_a"
  Mz_a/1 -> Mux/6  "Mz_a"
  Airdata/1 -> Bus Selector5/1
  chord/1 -> My_a/3
  span/1 -> Mz_a/3, Mx_a/3
  Fy_a(Side)/1 -> Mux/2  "Fy_a"
  Mux/1 -> FM_w/1
  Bus Selector3/2 -> Mz_a/1  "<Cn>"
  Bus Selector/3 -> Fz_a(Lift)/1  "<CL>"
  Product1/1 -> Fx_a(Drag)/2, Fy_a(Side)/2, Fz_a(Lift)/2, Mx_a/2, My_a/2, Mz_a/2  "qS"
  span1/1 -> Product1/2
  Bus Selector3/1 -> Mx_a/1  "<Cl>"
  Bus Selector5/1 -> Product1/1  "<q>"

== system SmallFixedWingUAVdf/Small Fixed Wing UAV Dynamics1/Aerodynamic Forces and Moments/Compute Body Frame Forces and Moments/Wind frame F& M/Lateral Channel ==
  beta : Inport
  Airspeed : Inport  Port=2
  dA : Inport  Port=3
  dR : Inport  Port=4
  p,q,r : Inport  Port=5
  Bus Creator : BusCreator  Inputs=3
  CY : Subsystem
  Cl : Subsystem
  Cn : Subsystem
  Lateral : Outport  VectorParamsAs1DForOutWhenUnconnected=off
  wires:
  Cl/1(Cl) -> Bus Creator/2  "Cl"
  p,q,r/1 -> Cn/4(p,q,r), Cl/4(p,q,r)
  Airspeed/1 -> Cn/5(Airspeed), Cl/5(Airspeed)
  dR/1 -> CY/2(dR), Cl/3(dR), Cn/3(dR)
  dA/1 -> Cl/2(dA), Cn/2(dA)
  beta/1 -> CY/1(beta), Cl/1(beta), Cn/1(beta)
  Cn/1(Cn) -> Bus Creator/3  "Cn"
  CY/1(CY) -> Bus Creator/1  "CY"
  Bus Creator/1 -> Lateral/1

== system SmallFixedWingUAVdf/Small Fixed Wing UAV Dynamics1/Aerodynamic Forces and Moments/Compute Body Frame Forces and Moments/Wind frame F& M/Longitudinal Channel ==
  alpha : Inport
  Airpseed : Inport  Port=2
  dE : Inport  Port=3
  dF : Inport  Port=4
  p,q,r : Inport  Port=5
  dR : Inport  Port=6
  Bus Creator : BusCreator  Inputs=3
  CD : Subsystem
  CL : Subsystem
  Cm : Subsystem
  Gain1 : Gain  Gain=-1
  Gain2 : Gain  Gain=-1
  Transfer Fcn : TransferFcn  Numerator=[1 0]  Denominator=[0.1 1]
  Longitudinal : Outport  VectorParamsAs1DForOutWhenUnconnected=off
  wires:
  Transfer Fcn/1 -> Cm/6(alpha_dot), CL/2(alpha_dot)
  Airpseed/1 -> Cm/5(Airspeed), CL/6(Airspeed)
  p,q,r/1 -> Cm/4(p,q,r), CL/5(p,q,r)
  dF/1 -> Cm/3(dF), CL/4(dF)
  Bus Creator/1 -> Longitudinal/1
  Cm/1(Cm) -> Bus Creator/3  "Cm"
  dE/1 -> Cm/2(dE), CD/2(dE), CL/3(dE)
  CL/1(CL) -> Gain1/1, CD/1(CL)  "CL"
  CD/1(CD) -> Gain2/1  "CD"
  alpha/1 -> Transfer Fcn/1, Cm/1(alpha), CL/1(alpha)
  dR/1 -> CD/3(dR)
  Gain1/1 -> Bus Creator/2  "CL"
  Gain2/1 -> Bus Creator/1  "CD"

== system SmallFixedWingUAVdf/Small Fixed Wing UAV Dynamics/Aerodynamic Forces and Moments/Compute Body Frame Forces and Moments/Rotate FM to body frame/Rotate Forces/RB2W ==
  aoa beta : Inport
  11 : Fcn  Expr=u[3]*u[4]
  12 : Fcn  Expr=u[2]
  13 : Fcn  Expr=u[1]*u[4]
  21 : Fcn  Expr=-u[3]*u[2]
  22 : Fcn  Expr=u[4]
  23 : Fcn  Expr=-u[1]*u[2]
  31 : Fcn  Expr=-u[1]
  32 : Fcn  Expr=0
  33 : Fcn  Expr=u[3]
  Mux : Mux  Inputs=2
  Mux3 : Mux  Inputs=9
  Reshape 9x1->3x3 : Reshape  OutputDimensionality=Customize  OutputDimensions=[3,3]
  sincos : Trigonometry  Operator=sincos
  Rw2b : Outport  VectorParamsAs1DForOutWhenUnconnected=off
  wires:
  Mux/1 -> 11/1, 21/1, 31/1, 12/1, 22/1, 32/1, 13/1, 23/1, 33/1
  aoa beta/1 -> sincos/1
  sincos/2 -> Mux/2
  sincos/1 -> Mux/1
  33/1 -> Mux3/9
  23/1 -> Mux3/8
  13/1 -> Mux3/7
  32/1 -> Mux3/6
  22/1 -> Mux3/5
  12/1 -> Mux3/4
  31/1 -> Mux3/3
  21/1 -> Mux3/2
  11/1 -> Mux3/1
  Reshape 9x1->3x3/1 -> Rw2b/1
  Mux3/1 -> Reshape 9x1->3x3/1

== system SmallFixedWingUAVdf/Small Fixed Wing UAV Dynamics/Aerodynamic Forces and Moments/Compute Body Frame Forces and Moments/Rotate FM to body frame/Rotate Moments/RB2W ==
  aoa beta : Inport
  11 : Fcn  Expr=u[3]*u[4]
  12 : Fcn  Expr=u[2]
  13 : Fcn  Expr=u[1]*u[4]
  21 : Fcn  Expr=-u[3]*u[2]
  22 : Fcn  Expr=u[4]
  23 : Fcn  Expr=-u[1]*u[2]
  31 : Fcn  Expr=-u[1]
  32 : Fcn  Expr=0
  33 : Fcn  Expr=u[3]
  Mux : Mux  Inputs=2
  Mux3 : Mux  Inputs=9
  Reshape 9x1->3x3 : Reshape  OutputDimensionality=Customize  OutputDimensions=[3,3]
  sincos : Trigonometry  Operator=sincos
  Rw2b : Outport  VectorParamsAs1DForOutWhenUnconnected=off
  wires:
  Mux/1 -> 11/1, 21/1, 31/1, 12/1, 22/1, 32/1, 13/1, 23/1, 33/1
  aoa beta/1 -> sincos/1
  sincos/2 -> Mux/2
  sincos/1 -> Mux/1
  33/1 -> Mux3/9
  23/1 -> Mux3/8
  13/1 -> Mux3/7
  32/1 -> Mux3/6
  22/1 -> Mux3/5
  12/1 -> Mux3/4
  31/1 -> Mux3/3
  21/1 -> Mux3/2
  11/1 -> Mux3/1
  Reshape 9x1->3x3/1 -> Rw2b/1
  Mux3/1 -> Reshape 9x1->3x3/1

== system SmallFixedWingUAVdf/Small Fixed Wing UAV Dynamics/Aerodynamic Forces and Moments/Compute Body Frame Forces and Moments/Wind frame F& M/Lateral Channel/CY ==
  beta : Inport
  dR : Inport  Port=2
  CYDr : Constant  Value=uav.aero.CYDr
  CYb : Constant  Value=uav.aero.CYb
  Product : Product  SaturateOnIntegerOverflow=on
  Product1 : Product  SaturateOnIntegerOverflow=on
  Sum2 : Sum  SaturateOnIntegerOverflow=on
  CY : Outport  VectorParamsAs1DForOutWhenUnconnected=off
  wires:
  Product1/1 -> Sum2/2
  dR/1 -> Product1/2
  CYDr/1 -> Product1/1
  Product/1 -> Sum2/1
  Sum2/1 -> CY/1
  beta/1 -> Product/2
  CYb/1 -> Product/1

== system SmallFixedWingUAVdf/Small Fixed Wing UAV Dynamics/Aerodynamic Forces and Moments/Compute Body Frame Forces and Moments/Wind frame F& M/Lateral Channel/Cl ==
  beta : Inport
  dA : Inport  Port=2
  dR : Inport  Port=3
  p,q,r : Inport  Port=4
  Airspeed : Inport  Port=5
  ClDa : Constant  Value=uav.aero.ClDa
  ClDr : Constant  Value=uav.aero.ClDr
  Clb : Constant  Value=uav.aero.Clb
  Product1 : Product  SaturateOnIntegerOverflow=on
  Product4 : Product  SaturateOnIntegerOverflow=on
  Product5 : Product  SaturateOnIntegerOverflow=on
  Sum : Sum  Inputs=+++++  SaturateOnIntegerOverflow=on
  roll factors : Subsystem
  Cl : Outport  VectorParamsAs1DForOutWhenUnconnected=off
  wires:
  roll factors/1(Clp) -> Sum/4
  Product5/1 -> Sum/2  "CldA"
  Airspeed/1 -> roll factors/2(Airspeed)
  p,q,r/1 -> roll factors/1(p,q,r)
  roll factors/2(Clr) -> Sum/5
  Product1/1 -> Sum/3  "Cldr"
  Product4/1 -> Sum/1  "Clb"
  Sum/1 -> Cl/1
  dR/1 -> Product1/2
  ClDr/1 -> Product1/1
  dA/1 -> Product5/2
  ClDa/1 -> Product5/1
  beta/1 -> Product4/2
  Clb/1 -> Product4/1

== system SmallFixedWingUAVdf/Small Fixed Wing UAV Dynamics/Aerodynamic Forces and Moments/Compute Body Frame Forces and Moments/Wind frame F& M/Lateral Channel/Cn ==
  beta : Inport
  dA : Inport  Port=2
  dR : Inport  Port=3
  p,q,r : Inport  Port=4
  Airspeed : Inport  Port=5
  CnDa : Constant  Value=uav.aero.CnDa
  CnDr : Constant  Value=uav.aero.CnDr
  Cnb : Constant  Value=uav.aero.Cnb
  Product1 : Product  SaturateOnIntegerOverflow=on
  Product4 : Product  SaturateOnIntegerOverflow=on
  Product5 : Product  SaturateOnIntegerOverflow=on
  Sum : Sum  Inputs=+++++  SaturateOnIntegerOverflow=on
  yaw factors : Subsystem
  Cn : Outport  VectorParamsAs1DForOutWhenUnconnected=off
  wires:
  Airspeed/1 -> yaw factors/2(Airspeed)
  p,q,r/1 -> yaw factors/1(p,q,r)
  Cnb/1 -> Product4/1
  beta/1 -> Product4/2
  CnDa/1 -> Product5/1
  Product5/1 -> Sum/2
  dA/1 -> Product5/2
  CnDr/1 -> Product1/1
  dR/1 -> Product1/2
  Sum/1 -> Cn/1
  Product1/1 -> Sum/3
  yaw factors/2(Cnr) -> Sum/5
  yaw factors/1(Cnp) -> Sum/4
  Product4/1 -> Sum/1

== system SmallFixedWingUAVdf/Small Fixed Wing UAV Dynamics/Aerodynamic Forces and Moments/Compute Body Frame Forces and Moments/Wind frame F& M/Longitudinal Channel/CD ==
  CL : Inport
  Apolar : Constant  Value=uav.aero.A1
  Apolar (A2) : Constant  Value=uav.aero.Apolar
  CD0 : Constant  Value=uav.aero.CD0
  Gain : Gain  Gain=-1  SaturateOnIntegerOverflow=on
  Math Function : Math  Operator=square  SignedPower=on
  Product : Product  SaturateOnIntegerOverflow=on
  Product1 : Product  SaturateOnIntegerOverflow=on
  Sum1 : Sum  Inputs=+++  SaturateOnIntegerOverflow=on
  CD : Outport  VectorParamsAs1DForOutWhenUnconnected=off
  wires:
  Gain/1 -> CD/1
  Apolar (A2)/1 -> Product/1
  Math Function/1 -> Product/2
  Product1/1 -> Sum1/3
  Product/1 -> Sum1/2
  CL/1 -> Math Function/1, Product1/1
  Sum1/1 -> Gain/1
  CD0/1 -> Sum1/1
  Apolar/1 -> Product1/2

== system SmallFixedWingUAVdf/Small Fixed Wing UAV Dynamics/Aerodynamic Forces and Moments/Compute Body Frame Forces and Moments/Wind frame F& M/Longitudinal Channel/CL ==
  alpha : Inport
  alpha_dot : Inport  Port=2
  dE : Inport  Port=3
  dF : Inport  Port=4
  p,q,r : Inport  Port=5
  Airspeed : Inport  Port=6
  CL0 : Constant  Value=uav.aero.CL0
  CLDe : Constant  Value=uav.aero.CLDe
  CLa : Constant  Value=uav.aero.CLa
  CLa_dot : Constant  Value=uav.aero.CLa_dot
  CmDe1 : Constant  Value=uav.aero.CLDf
  Lift due to pitch rate : Subsystem
  Product{1..2,4..5} (4 alike) : Product  SaturateOnIntegerOverflow=on
  Sum : Sum  Inputs=++++++  SaturateOnIntegerOverflow=on
  CL : Outport  VectorParamsAs1DForOutWhenUnconnected=off
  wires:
  CL0/1 -> Sum/1
  Airspeed/1 -> Lift due to pitch rate/2(Airspeed)
  p,q,r/1 -> Lift due to pitch rate/1(p,q,r)
  Lift due to pitch rate/1(CLq) -> Sum/6
  Product2/1 -> Sum/5
  Product1/1 -> Sum/4
  Product5/1 -> Sum/3
  CmDe1/1 -> Product2/1
  dF/1 -> Product2/2
  Sum/1 -> CL/1
  dE/1 -> Product1/2
  CLDe/1 -> Product1/1
  alpha_dot/1 -> Product5/2
  CLa_dot/1 -> Product5/1
  alpha/1 -> Product4/2
  CLa/1 -> Product4/1
  Product4/1 -> Sum/2

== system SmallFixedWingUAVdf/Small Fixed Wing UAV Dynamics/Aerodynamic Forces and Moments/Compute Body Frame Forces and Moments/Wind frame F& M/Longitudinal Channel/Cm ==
  alpha : Inport
  dE : Inport  Port=2
  dF : Inport  Port=3
  p,q,r : Inport  Port=4
  Cm0 : Constant  Value=uav.aero.Cm0
  CmDe : Constant  Value=uav.aero.CmDe
  CmDf : Constant  Value=uav.aero.CmDf
  Cma : Constant  Value=uav.aero.Cma
  Cma1 : Constant  Value=uav.aero.Cmq
  Get q : Selector  InputPortWidth=3  IndexOptions=Index vector (dialog)  Indices=2  OutputSizes=[(-2)]
  Product1 : Product  Inputs=***/  SaturateOnIntegerOverflow=on
  Product2 : Product  SaturateOnIntegerOverflow=on
  Product3 : Product  SaturateOnIntegerOverflow=on
  Product4 : Product  SaturateOnIntegerOverflow=on
  Sum : Sum  Inputs=+++++  SaturateOnIntegerOverflow=on
  chord : Constant  Value=uav.geometry.chord
  elarm : Constant  Value=uav.geometry.elarm
  Cm : Outport  VectorParamsAs1DForOutWhenUnconnected=off
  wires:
  chord/1 -> Product1/4
  elarm/1 -> Product1/3
  Get q/1 -> Product3/2
  Product3/1 -> Sum/5  "cmq"
  p,q,r/1 -> Get q/1
  Cma1/1 -> Product3/1
  Product1/1 -> Sum/3  "cmde"
  Product4/1 -> Sum/2  "cma"
  Sum/1 -> Cm/1  "total"
  dE/1 -> Product1/2
  CmDe/1 -> Product1/1
  alpha/1 -> Product4/2
  Cma/1 -> Product4/1
  dF/1 -> Product2/2
  CmDf/1 -> Product2/1
  Product2/1 -> Sum/4  "cmdf"
  Cm0/1 -> Sum/1  "cm0"

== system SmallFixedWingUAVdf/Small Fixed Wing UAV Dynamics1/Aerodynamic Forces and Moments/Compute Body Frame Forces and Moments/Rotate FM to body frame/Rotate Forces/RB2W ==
  aoa beta : Inport
  11 : Fcn  Expr=u[3]*u[4]
  12 : Fcn  Expr=u[2]
  13 : Fcn  Expr=u[1]*u[4]
  21 : Fcn  Expr=-u[3]*u[2]
  22 : Fcn  Expr=u[4]
  23 : Fcn  Expr=-u[1]*u[2]
  31 : Fcn  Expr=-u[1]
  32 : Fcn  Expr=0
  33 : Fcn  Expr=u[3]
  Mux : Mux  Inputs=2
  Mux3 : Mux  Inputs=9
  Reshape 9x1->3x3 : Reshape  OutputDimensionality=Customize  OutputDimensions=[3,3]
  sincos : Trigonometry  Operator=sincos
  Rw2b : Outport  VectorParamsAs1DForOutWhenUnconnected=off
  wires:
  Mux/1 -> 11/1, 21/1, 31/1, 12/1, 22/1, 32/1, 13/1, 23/1, 33/1
  aoa beta/1 -> sincos/1
  sincos/2 -> Mux/2
  sincos/1 -> Mux/1
  33/1 -> Mux3/9
  23/1 -> Mux3/8
  13/1 -> Mux3/7
  32/1 -> Mux3/6
  22/1 -> Mux3/5
  12/1 -> Mux3/4
  31/1 -> Mux3/3
  21/1 -> Mux3/2
  11/1 -> Mux3/1
  Reshape 9x1->3x3/1 -> Rw2b/1
  Mux3/1 -> Reshape 9x1->3x3/1

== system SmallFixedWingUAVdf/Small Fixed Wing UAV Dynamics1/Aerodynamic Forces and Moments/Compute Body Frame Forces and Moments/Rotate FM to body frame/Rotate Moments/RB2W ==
  aoa beta : Inport
  11 : Fcn  Expr=u[3]*u[4]
  12 : Fcn  Expr=u[2]
  13 : Fcn  Expr=u[1]*u[4]
  21 : Fcn  Expr=-u[3]*u[2]
  22 : Fcn  Expr=u[4]
  23 : Fcn  Expr=-u[1]*u[2]
  31 : Fcn  Expr=-u[1]
  32 : Fcn  Expr=0
  33 : Fcn  Expr=u[3]
  Mux : Mux  Inputs=2
  Mux3 : Mux  Inputs=9
  Reshape 9x1->3x3 : Reshape  OutputDimensionality=Customize  OutputDimensions=[3,3]
  sincos : Trigonometry  Operator=sincos
  Rw2b : Outport  VectorParamsAs1DForOutWhenUnconnected=off
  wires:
  Mux/1 -> 11/1, 21/1, 31/1, 12/1, 22/1, 32/1, 13/1, 23/1, 33/1
  aoa beta/1 -> sincos/1
  sincos/2 -> Mux/2
  sincos/1 -> Mux/1
  33/1 -> Mux3/9
  23/1 -> Mux3/8
  13/1 -> Mux3/7
  32/1 -> Mux3/6
  22/1 -> Mux3/5
  12/1 -> Mux3/4
  31/1 -> Mux3/3
  21/1 -> Mux3/2
  11/1 -> Mux3/1
  Reshape 9x1->3x3/1 -> Rw2b/1
  Mux3/1 -> Reshape 9x1->3x3/1

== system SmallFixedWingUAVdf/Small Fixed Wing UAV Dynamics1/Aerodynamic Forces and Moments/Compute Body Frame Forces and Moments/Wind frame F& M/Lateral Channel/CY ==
  beta : Inport
  dR : Inport  Port=2
  CYDr : Constant  Value=uav.aero.CYDr
  CYb : Constant  Value=uav.aero.CYb
  Product : Product  SaturateOnIntegerOverflow=on
  Product1 : Product  SaturateOnIntegerOverflow=on
  Sum2 : Sum  SaturateOnIntegerOverflow=on
  CY : Outport  VectorParamsAs1DForOutWhenUnconnected=off
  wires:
  Product1/1 -> Sum2/2
  dR/1 -> Product1/2
  CYDr/1 -> Product1/1
  Product/1 -> Sum2/1
  Sum2/1 -> CY/1
  beta/1 -> Product/2
  CYb/1 -> Product/1

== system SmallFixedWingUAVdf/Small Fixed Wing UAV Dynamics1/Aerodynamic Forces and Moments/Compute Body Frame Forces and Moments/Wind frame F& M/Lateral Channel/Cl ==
  beta : Inport
  dA : Inport  Port=2
  dR : Inport  Port=3
  p,q,r : Inport  Port=4
  Airspeed : Inport  Port=5
  ClDa : Constant  Value=uav.aero.ClDa
  ClDr : Constant  Value=uav.aero.ClDr
  Clb : Constant  Value=uav.aero.Clb
  Product1 : Product  SaturateOnIntegerOverflow=on
  Product4 : Product  SaturateOnIntegerOverflow=on
  Product5 : Product  SaturateOnIntegerOverflow=on
  Sum : Sum  Inputs=+++++  SaturateOnIntegerOverflow=on
  roll and yaw factors : Subsystem
  Cl : Outport  VectorParamsAs1DForOutWhenUnconnected=off
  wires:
  roll and yaw factors/1(Clp) -> Sum/4
  Product5/1 -> Sum/2  "Clda"
  Airspeed/1 -> roll and yaw factors/2(Airspeed)
  p,q,r/1 -> roll and yaw factors/1(p,q,r)
  roll and yaw factors/2(Clr) -> Sum/5
  Product1/1 -> Sum/3  "Cldr"
  Product4/1 -> Sum/1  "Clb"
  Sum/1 -> Cl/1
  dR/1 -> Product1/2
  ClDr/1 -> Product1/1
  dA/1 -> Product5/2
  ClDa/1 -> Product5/1
  beta/1 -> Product4/2
  Clb/1 -> Product4/1

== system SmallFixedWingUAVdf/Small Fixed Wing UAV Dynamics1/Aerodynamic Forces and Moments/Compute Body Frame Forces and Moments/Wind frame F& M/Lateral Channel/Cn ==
  beta : Inport
  dA : Inport  Port=2
  dR : Inport  Port=3
  p,q,r : Inport  Port=4
  Airspeed : Inport  Port=5
  CnDa : Constant  Value=uav.aero.CnDa
  CnDr : Constant  Value=uav.aero.CnDr
  Cnb : Constant  Value=uav.aero.Cnb
  Product1 : Product  SaturateOnIntegerOverflow=on
  Product4 : Product  SaturateOnIntegerOverflow=on
  Product5 : Product  SaturateOnIntegerOverflow=on
  Sum : Sum  Inputs=+++++  SaturateOnIntegerOverflow=on
  yaw factors : Subsystem
  Cn : Outport  VectorParamsAs1DForOutWhenUnconnected=off
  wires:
  Airspeed/1 -> yaw factors/2(Airspeed)
  p,q,r/1 -> yaw factors/1(p,q,r)
  Cnb/1 -> Product4/1
  beta/1 -> Product4/2
  CnDa/1 -> Product5/1
  Product5/1 -> Sum/2  "Cnda"
  dA/1 -> Product5/2
  CnDr/1 -> Product1/1
  dR/1 -> Product1/2
  Sum/1 -> Cn/1
  Product1/1 -> Sum/3  "Cndr"
  yaw factors/2(Cnr) -> Sum/5
  yaw factors/1(Cnp) -> Sum/4
  Product4/1 -> Sum/1  "Cnb"
